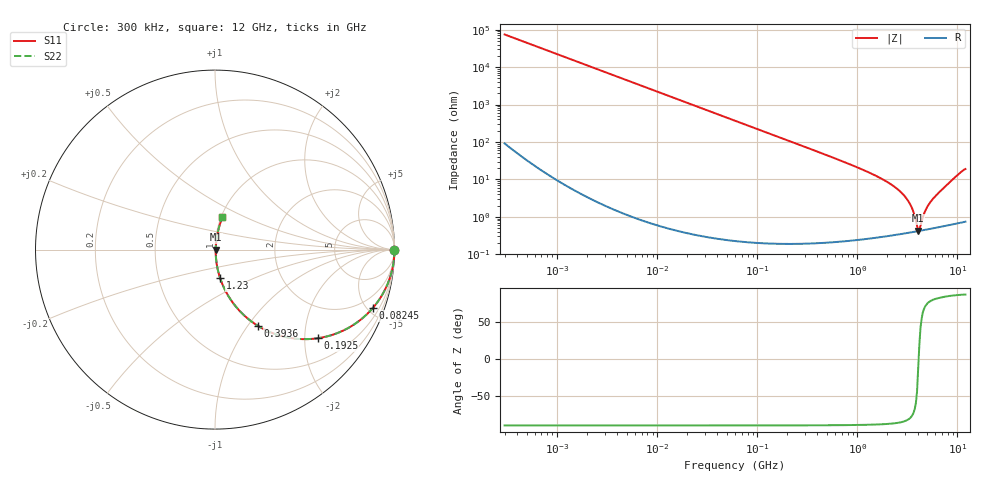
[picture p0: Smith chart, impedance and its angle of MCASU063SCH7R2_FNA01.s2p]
! MCASU063SCH7R2_FNA01  S-PARAMETER MODEL  ( General Type )
! Model Generated by TAIYO YUDEN Corporation (http://www.ty-top.com)
! Version 1.0
! TAIYO YUDEN Control No. 130801
! Copyright(c) 2013 TAIYO YUDEN CO.,LTD. All Rights Reserved.
! Product Description (link to TY-COMPAS)
! https://ds.yuden.co.jp/TYCOMPAS/or/detail?pn=MCASU063SCH7R2DFNA01&u=M
! Products Name : Multilayer Ceramic Capacitors
! Characteristics :
!  Capacitance : 7.2 pF , Rated Voltage : 50V , TCC : CH / C0H
!  Case Size : 0.6 x 0.3 / 0.024 x 0.012 [mm/inch] , Thickness : 0.3 / 0.012 [mm/inch]
!  (Conditions: Temperature = 25 degC , DC Bias Current/Voltage = 0A / 0V)
! External Node Assignments :
!  1  o---| |---o  2
! GND o---------o GND
! Frequency Range : 0.3MHz  -  12000MHz  [ 401 STEP ]
# MHz S RI R 50
! Freq[MHz].  S11 Real  S11 Imag  S21 Real  S21 Imag  S12 Real  S12 Imag  S22 Real  S22 Imag
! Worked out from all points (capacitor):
!   401 points, 300 kHz to 12 GHz, reference 50 ohm
!   read as one part in series: C = 7.14 pF near 316.3 kHz
!   lowest |Z| = 428 mohm at 4.05 GHz (marker M1)
!   series resonance near 4.095 GHz, so ESL is about 210 pH
!   S11 on the Smith chart (normalised r, x): 300 kHz: open; 82.45 MHz: 1.00, -5.40; 192.5 MHz: 1.00, -2.31; 393.6 MHz: 1.00, -1.12; 1.23 GHz: 1.01, -0.33; 12 GHz: 1.01, +0.38
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0.3  1 -0.00135  3.47e-06 0.00135  3.47e-06 0.00135  1 -0.00135
1.769972  0.9999 -0.00794  6.56e-05 0.00794  6.56e-05 0.00794  0.9999 -0.00794
10.44266  0.9978 -0.0468  0.0022 0.0468  0.0022 0.0468  0.9978 -0.0468
27.10171  0.9854 -0.1199  0.0146 0.1199  0.0146 0.1199  0.9854 -0.1199
60  0.9322 -0.251  0.0678 0.251  0.0678 0.251  0.9322 -0.251
82.45425  0.8793 -0.3254  0.1207 0.3254  0.1207 0.3254  0.8793 -0.3254
192.4766  0.5715 -0.494  0.4285 0.494  0.4285 0.494  0.5715 -0.494
353.9943  0.2813 -0.4481  0.7187 0.4481  0.7187 0.4481  0.2813 -0.4481
393.5654  0.2401 -0.4254  0.7599 0.4254  0.7599 0.4254  0.2401 -0.4254
651.0506  0.1017 -0.299  0.8983 0.299  0.8983 0.299  0.1017 -0.299
1229.528  0.0288 -0.1597  0.9712 0.1597  0.9712 0.1597  0.0288 -0.1597
2088.533  0.00923 -0.078  0.9908 0.078  0.9908 0.078  0.00923 -0.078
2650.866  0.00577 -0.0484  0.9942 0.0484  0.9942 0.0484  0.00577 -0.0484
3190.978  0.00445 -0.0272  0.9955 0.0272  0.9955 0.0272  0.00445 -0.0272
3547.679  0.00414 -0.0155  0.9959 0.0155  0.9959 0.0155  0.00414 -0.0155
3944.255  0.00411 -0.00403  0.9959 0.00403  0.9959 0.00403  0.00411 -0.00403
4050.141  0.00415 -0.000981  0.9959 0.000981  0.9959 0.000981  0.00415 -0.000981
4270.516  0.00427 0.00384  0.9957 -0.00384  0.9957 -0.00384  0.00427 0.00384
4875.354  0.00478 0.0155  0.9952 -0.0155  0.9952 -0.0155  0.00478 0.0155
5715.274  0.00584 0.0303  0.9942 -0.0303  0.9942 -0.0303  0.00584 0.0303
8966.534  0.0161 0.0983  0.9839 -0.0983  0.9839 -0.0983  0.0161 0.0983
12000  0.0412 0.1802  0.9588 -0.1802  0.9588 -0.1802  0.0412 0.1802
